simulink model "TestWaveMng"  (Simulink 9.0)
settings: Solver=FixedStepDiscrete  StartTime=0.0  StopTime=10.0  FixedStep=Tstep  RelTol=1e-3  EnableMultiTasking=on
PreLoadFcn:
  | TestWaveMng.TestWaveMng_init();
InitFcn:
  | TestWaveMng.TestWaveMng_init();
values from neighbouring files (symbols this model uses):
  Tstep = 0.00005    (= 5e-05)    [TestWaveMng_init.m]    (also in TestOrthOscObjO_init.m = 0.0005)
libraries: lib_WaveMng x16

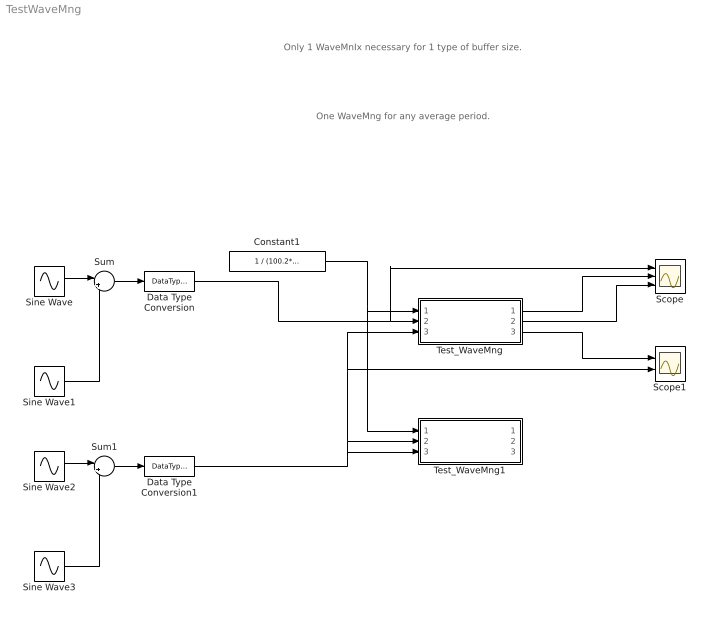
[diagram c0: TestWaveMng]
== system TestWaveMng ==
  note: One WaveMng for any average period.
  note: Only 1 WaveMnIx necessary for 1 type of buffer size.
  Constant1 : Constant  Value=1 / (100.2* Tstep)  OutDataTypeStr=single
  Data Type Conversion : DataTypeConversion  OutDataTypeStr=single
  Data Type Conversion1 : DataTypeConversion  OutDataTypeStr=single
  Scope : Scope  NumInputPorts=3
  Scope1 : Scope  NumInputPorts=2
  Sine Wave : Sin  Amplitude=1.676  Frequency=100.2*2*pi  SampleTime=Tstep
  Sine Wave1 : Sin  Amplitude=0.5  Frequency=300.6*2*pi  SampleTime=Tstep
  Sine Wave2 : Sin  Amplitude=1.676  Frequency=104  SampleTime=Tstep
  Sine Wave3 : Sin  Amplitude=0.2  Frequency=15*104  SampleTime=Tstep
  Sum : Sum  Inputs=|++
  Sum1 : Sum  Inputs=|++
  Test_WaveMng : Subsystem  TreatAsAtomicUnit=on
  Test_WaveMng1 : Subsystem  TreatAsAtomicUnit=on
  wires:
  Sine Wave/1 -> Sum/1
  Sine Wave1/1 -> Sum/2
  Sum/1 -> Data Type Conversion/1
  Sine Wave2/1 -> Sum1/1
  Sine Wave3/1 -> Sum1/2
  Sum1/1 -> Data Type Conversion1/1
  Constant1/1 -> Test_WaveMng1/1(In1), Test_WaveMng/1(In1)
  Data Type Conversion/1 -> Scope/1, Test_WaveMng/2(In2)
  Data Type Conversion1/1 -> Test_WaveMng1/3(In3), Test_WaveMng1/2(In2), Scope1/2, Test_WaveMng/3(In3)
  Test_WaveMng/1(Out1) -> Scope/2
  Test_WaveMng/2(Out2) -> Scope/3
  Test_WaveMng/3(Out3) -> Scope1/1

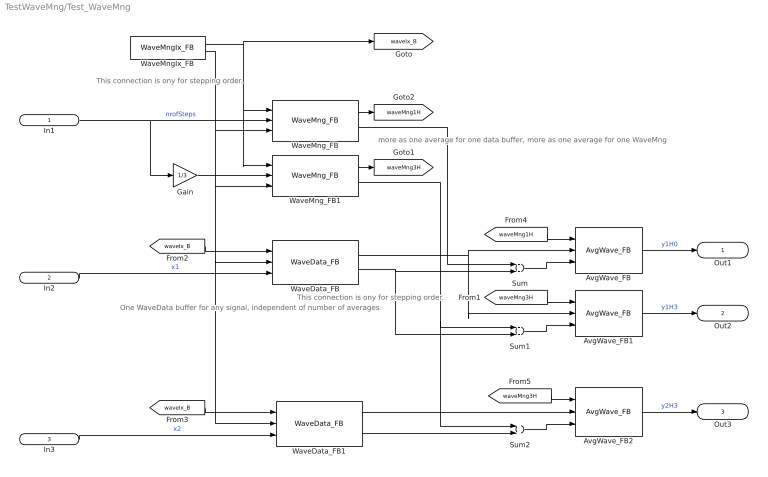
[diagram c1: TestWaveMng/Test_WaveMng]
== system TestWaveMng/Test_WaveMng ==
  note: more as one average for one data buffer, more as one average for one WaveMng
  note: This connection is ony for stepping order.
  note: One WaveData buffer for any signal, independent of number of averages
  note: This connection is ony for stepping order.
  In1 : Inport  OutDataTypeStr=single  PortDimensions=1
  In2 : Inport  Port=2  OutDataTypeStr=single  PortDimensions=1
  In3 : Inport  Port=3  OutDataTypeStr=single  PortDimensions=1
  AvgWave_FB : lib_WaveMng/AvgWave_FB  identObj=1
  AvgWave_FB1 : lib_WaveMng/AvgWave_FB  identObj=1
  AvgWave_FB2 : lib_WaveMng/AvgWave_FB  identObj=1
  Gain : Gain  Gain=1/3
  Sum : Sum
  Sum1 : Sum
  Sum2 : Sum
  WaveData_FB : lib_WaveMng/WaveData_FB  identObj=1  size=1024
  WaveData_FB1 : lib_WaveMng/WaveData_FB  identObj=1  size=1024
  WaveMngIx_FB : lib_WaveMng/WaveMngIx_FB  identObj=1  size=1024  Tstep=Tstep
  WaveMng_FB : lib_WaveMng/WaveMng_FB  identObj=1
  WaveMng_FB1 : lib_WaveMng/WaveMng_FB  identObj=1
  Out1 : Outport  OutDataTypeStr=single  PortDimensions=1
  Out2 : Outport  Port=2  OutDataTypeStr=single  PortDimensions=1
  Out3 : Outport  Port=3  OutDataTypeStr=single  PortDimensions=1
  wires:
  Gain/1 -> WaveMng_FB1/2
  In1/1 -> WaveMng_FB/2, Gain/1  "nrofSteps"
  WaveMng_FB1/1 -> [waveMng3H]
  WaveMng_FB/1 -> [waveMng1H]
  In2/1 -> WaveData_FB/3  "x1"
  WaveData_FB/1 -> AvgWave_FB1/2, AvgWave_FB/2
  AvgWave_FB/1 -> Out1/1  "y1H0"
  AvgWave_FB1/1 -> Out2/1  "y1H3"
  In3/1 -> WaveData_FB1/3  "x2"
  AvgWave_FB2/1 -> Out3/1  "y2H3"
  WaveData_FB1/1 -> AvgWave_FB2/2
  [waveIx_B] -> WaveData_FB/1
  [waveIx_B] -> WaveData_FB1/1
  [waveMng1H] -> AvgWave_FB/1
  [waveMng3H] -> AvgWave_FB2/1
  [waveMng3H] -> AvgWave_FB1/1
  WaveMngIx_FB/2 -> WaveMng_FB/3, WaveData_FB1/2, WaveData_FB/2, WaveMng_FB1/3
  WaveMngIx_FB/1 -> [waveIx_B], WaveMng_FB/1, WaveMng_FB1/1
  Sum/1 -> AvgWave_FB/3
  Sum2/1 -> AvgWave_FB2/3
  Sum1/1 -> AvgWave_FB1/3
  WaveData_FB/2 -> Sum1/2, Sum/2
  WaveMng_FB/2 -> Sum/1
  WaveMng_FB1/2 -> Sum2/1, Sum1/1
  WaveData_FB1/2 -> Sum2/2

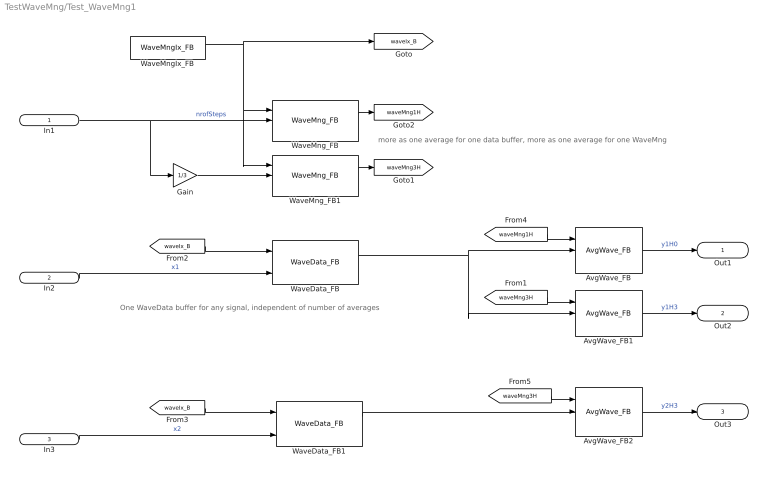
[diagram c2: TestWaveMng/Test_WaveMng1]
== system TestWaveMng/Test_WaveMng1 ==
  note: more as one average for one data buffer, more as one average for one WaveMng
  note: One WaveData buffer for any signal, independent of number of averages
  In1 : Inport  OutDataTypeStr=single  PortDimensions=1
  In2 : Inport  Port=2  OutDataTypeStr=single  PortDimensions=1
  In3 : Inport  Port=3  OutDataTypeStr=single  PortDimensions=1
  AvgWave_FB : lib_WaveMng/AvgWave_FB  identObj=1
  AvgWave_FB1 : lib_WaveMng/AvgWave_FB  identObj=1
  AvgWave_FB2 : lib_WaveMng/AvgWave_FB  identObj=1
  Gain : Gain  Gain=1/3
  WaveData_FB : lib_WaveMng/WaveData_FB  identObj=1  size=1024
  WaveData_FB1 : lib_WaveMng/WaveData_FB  identObj=1  size=1024
  WaveMngIx_FB : lib_WaveMng/WaveMngIx_FB  identObj=1  size=1024  Tstep=Tstep
  WaveMng_FB : lib_WaveMng/WaveMng_FB  identObj=1
  WaveMng_FB1 : lib_WaveMng/WaveMng_FB  identObj=1
  Out1 : Outport  OutDataTypeStr=single  PortDimensions=1
  Out2 : Outport  Port=2  OutDataTypeStr=single  PortDimensions=1
  Out3 : Outport  Port=3  OutDataTypeStr=single  PortDimensions=1
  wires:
  Gain/1 -> WaveMng_FB1/2
  In1/1 -> WaveMng_FB/2, Gain/1  "nrofSteps"
  WaveMng_FB1/1 -> [waveMng3H]
  WaveMng_FB/1 -> [waveMng1H]
  In2/1 -> WaveData_FB/3  "x1"
  WaveData_FB/1 -> AvgWave_FB1/2, AvgWave_FB/2
  AvgWave_FB/1 -> Out1/1  "y1H0"
  AvgWave_FB1/1 -> Out2/1  "y1H3"
  In3/1 -> WaveData_FB1/3  "x2"
  AvgWave_FB2/1 -> Out3/1  "y2H3"
  WaveData_FB1/1 -> AvgWave_FB2/2
  [waveIx_B] -> WaveData_FB/1
  [waveIx_B] -> WaveData_FB1/1
  [waveMng1H] -> AvgWave_FB/1
  [waveMng3H] -> AvgWave_FB2/1
  [waveMng3H] -> AvgWave_FB1/1
  WaveMngIx_FB/1 -> [waveIx_B], WaveMng_FB/1, WaveMng_FB1/1
